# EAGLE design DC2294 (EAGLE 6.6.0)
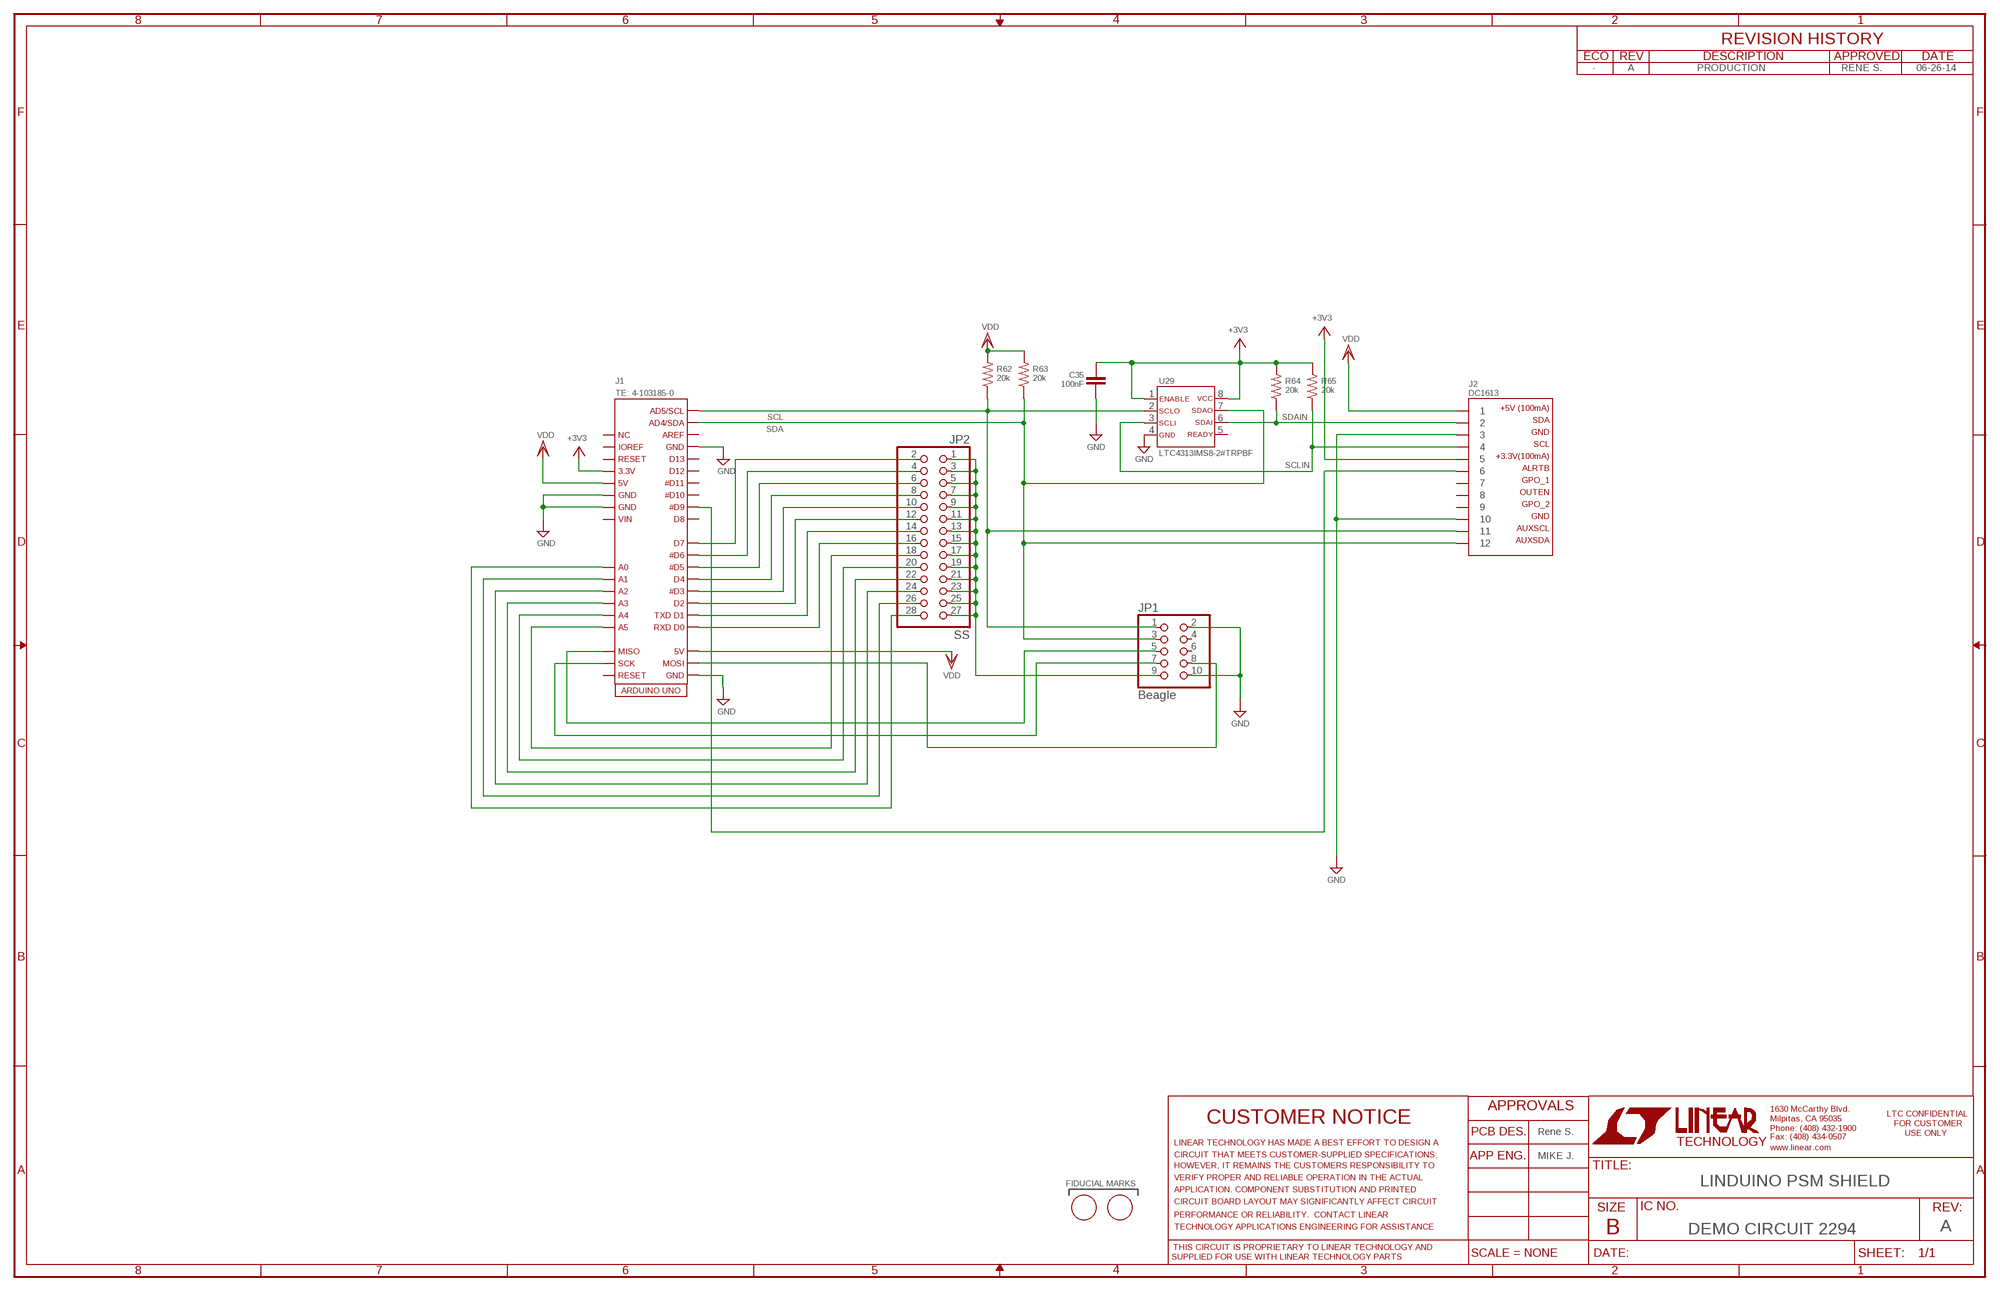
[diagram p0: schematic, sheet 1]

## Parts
C35  100nF  CC0603_BOX  [C0603_BOX]
FID1  FIDUCIAL  [FIDUCIAL_1MM]
FID2  FIDUCIAL  [FIDUCIAL_1MM]
J1  TE: 4-103185-0  ARDUINO_UNO_MINI_SHIELD_SPIFL  [ADRUINO_UNO_MINI_SHIELD_SPI_NOETH]
J2  DC1613  CONN_DC1613  [CONN_DC1613]
JP1  Beagle  PINHD-2X5  [2X05]
JP2  SS  PINHD-2X14  [2X14]
R62  20k  RR0603_BOX  [R0603_BOX]
R63  20k  RR0603_BOX  [R0603_BOX]
R64  20k  RR0603_BOX  [R0603_BOX]
R65  20k  RR0603_BOX  [R0603_BOX]
U29  LTC4313IMS8-2#TRPBF  LTC4313CMS8  [MSOP-8]

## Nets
+3V3: C35.1 J1.3V3 J2.5 R64.2 R65.2 U29.1 U29.8
GND: C35.2 J1.GND1 J1.GND2 J1.GND3 J1.GND4 J2.3 J2.10 JP1.2 JP1.10 U29.4
J1-A: J1.A0 JP2.28
N$1: J1.MISO JP1.5
N$2: J1.MOSI JP1.8
N$3: J1.SCK JP1.7
N$4: J1.D7 JP2.2
N$5: J1.D6 JP2.4
N$6: J1.D5 JP2.6
N$7: J1.D4 JP2.8
N$8: J1.D3 JP2.10
N$9: J1.D2 JP2.12
N$10: J1.D1 JP2.14
N$11: J1.D0 JP2.16
N$12: J1.A5 JP2.18
N$13: J1.A4 JP2.20
N$14: J1.A3 JP2.22
N$15: J1.A2 JP2.24
N$16: J1.A1 JP2.26
N$18: JP1.9 JP2.1 JP2.3 JP2.5 JP2.7 JP2.9 JP2.11 JP2.13 JP2.15 JP2.17 JP2.19 JP2.21 JP2.23 JP2.25 JP2.27
N$19: J1.D9 J2.6
SCL: J1.SCL J2.11 JP1.1 R62.1 U29.2
SCLIN: J2.4 R65.1 U29.3
SDA: J1.SDA J2.12 JP1.3 R63.1 U29.7
SDAIN: J2.2 R64.1 U29.6
VDD: J1.5V J1.5V1 J2.1 R62.2 R63.2
Unconnected: J1.D8 J1.D10 J1.D11 J1.D12 J1.D13 J1.NC J1.REF J1.RST1 J1.RST2 J1.VIN J1.VIO J2.7 J2.8 J2.9 JP1.4 JP1.6 U29.5

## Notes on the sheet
- A | PRODUCTION | RENE S. | 06-26-14
- Rene S.
- MIKE J.
- FIDUCIAL MARKS | LINDUINO PSM SHIELD
- DEMO CIRCUIT 2294 | A

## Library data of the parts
C35 = kalin:C: CAPACITOR, European symbol
FID1 FID2 = kalin:FIDUCIAL: For use by pick and place machines to calibrate the vision/machine, 1mm
J1 = kalin:ARDUINO_UNO_MINI_SHIELD_SPI: Arduino UNO Mini Shield With SPI
J2 = kalin:CONN_DC1613: Connector for LT DC1613 USB Dongle
JP1 = pinhead:PINHD-2X5: PIN HEADER
JP2 = pinhead:PINHD-2X14: PIN HEADER
R62-R65 = kalin:R: RESISTOR, American symbol
U29 = kalin:LTC4313: 2-Wire Bus Buffers with High Noise Margin

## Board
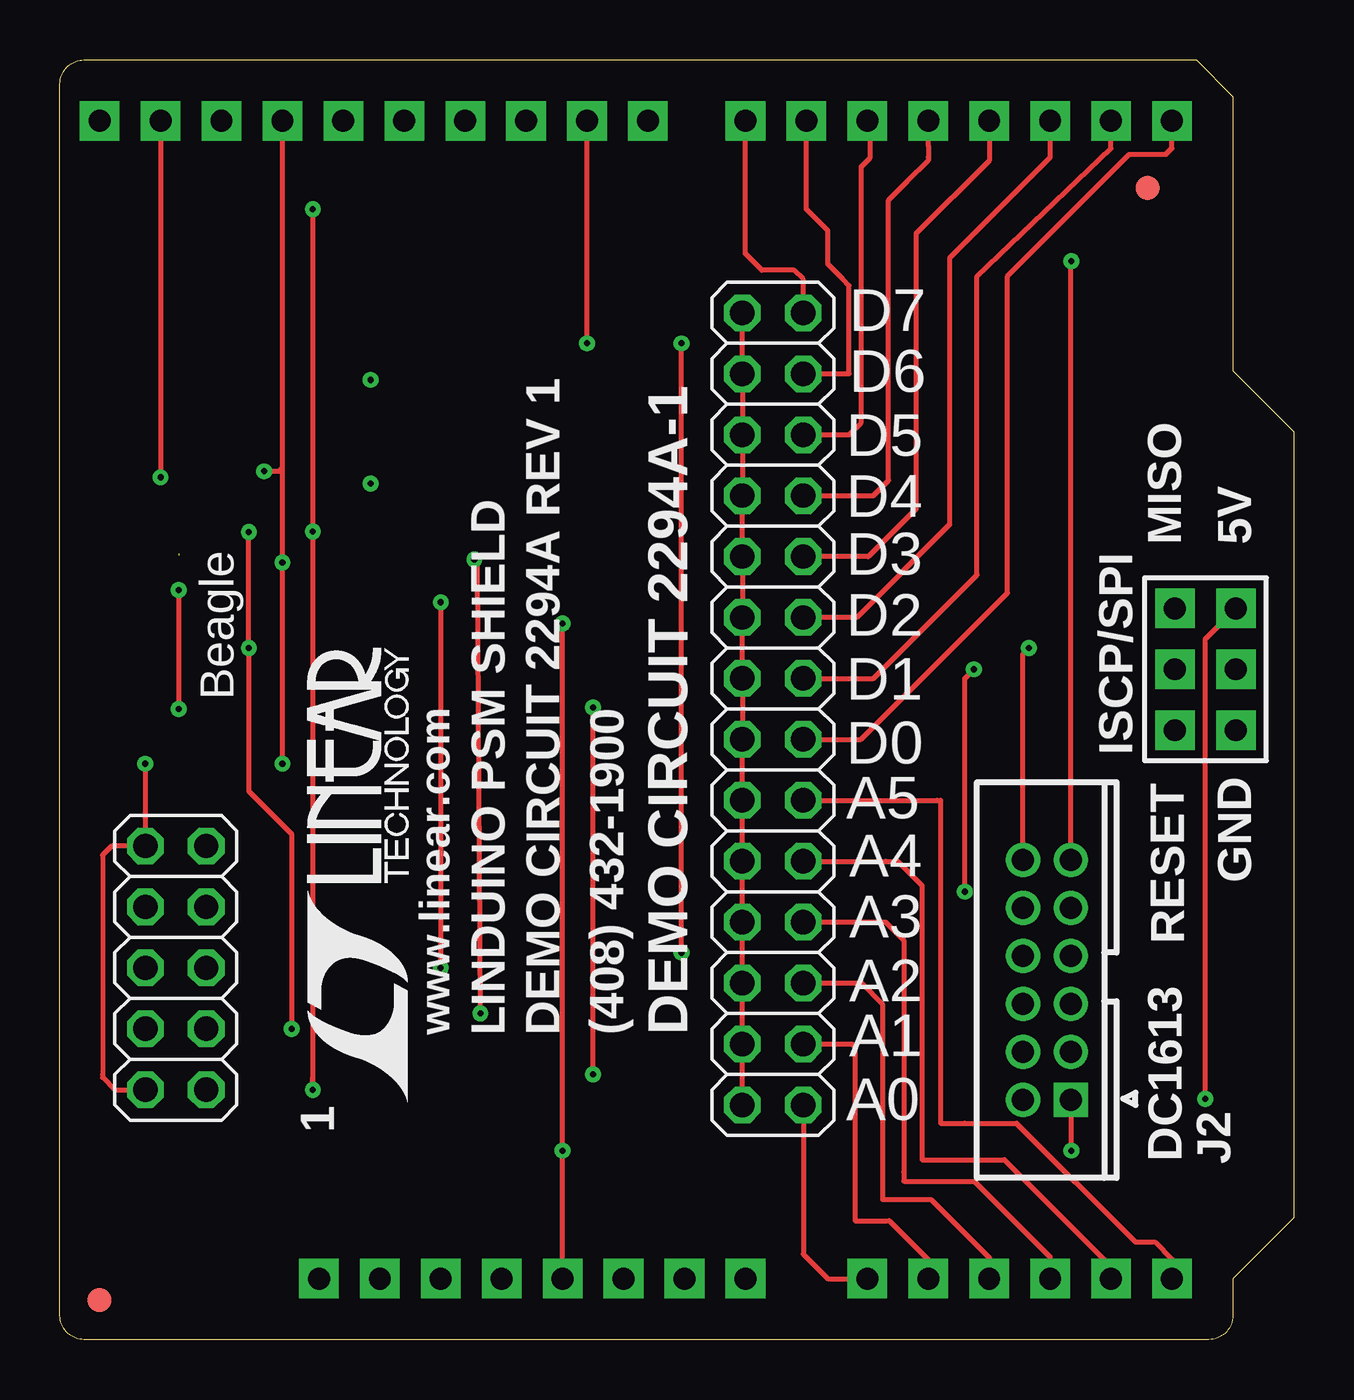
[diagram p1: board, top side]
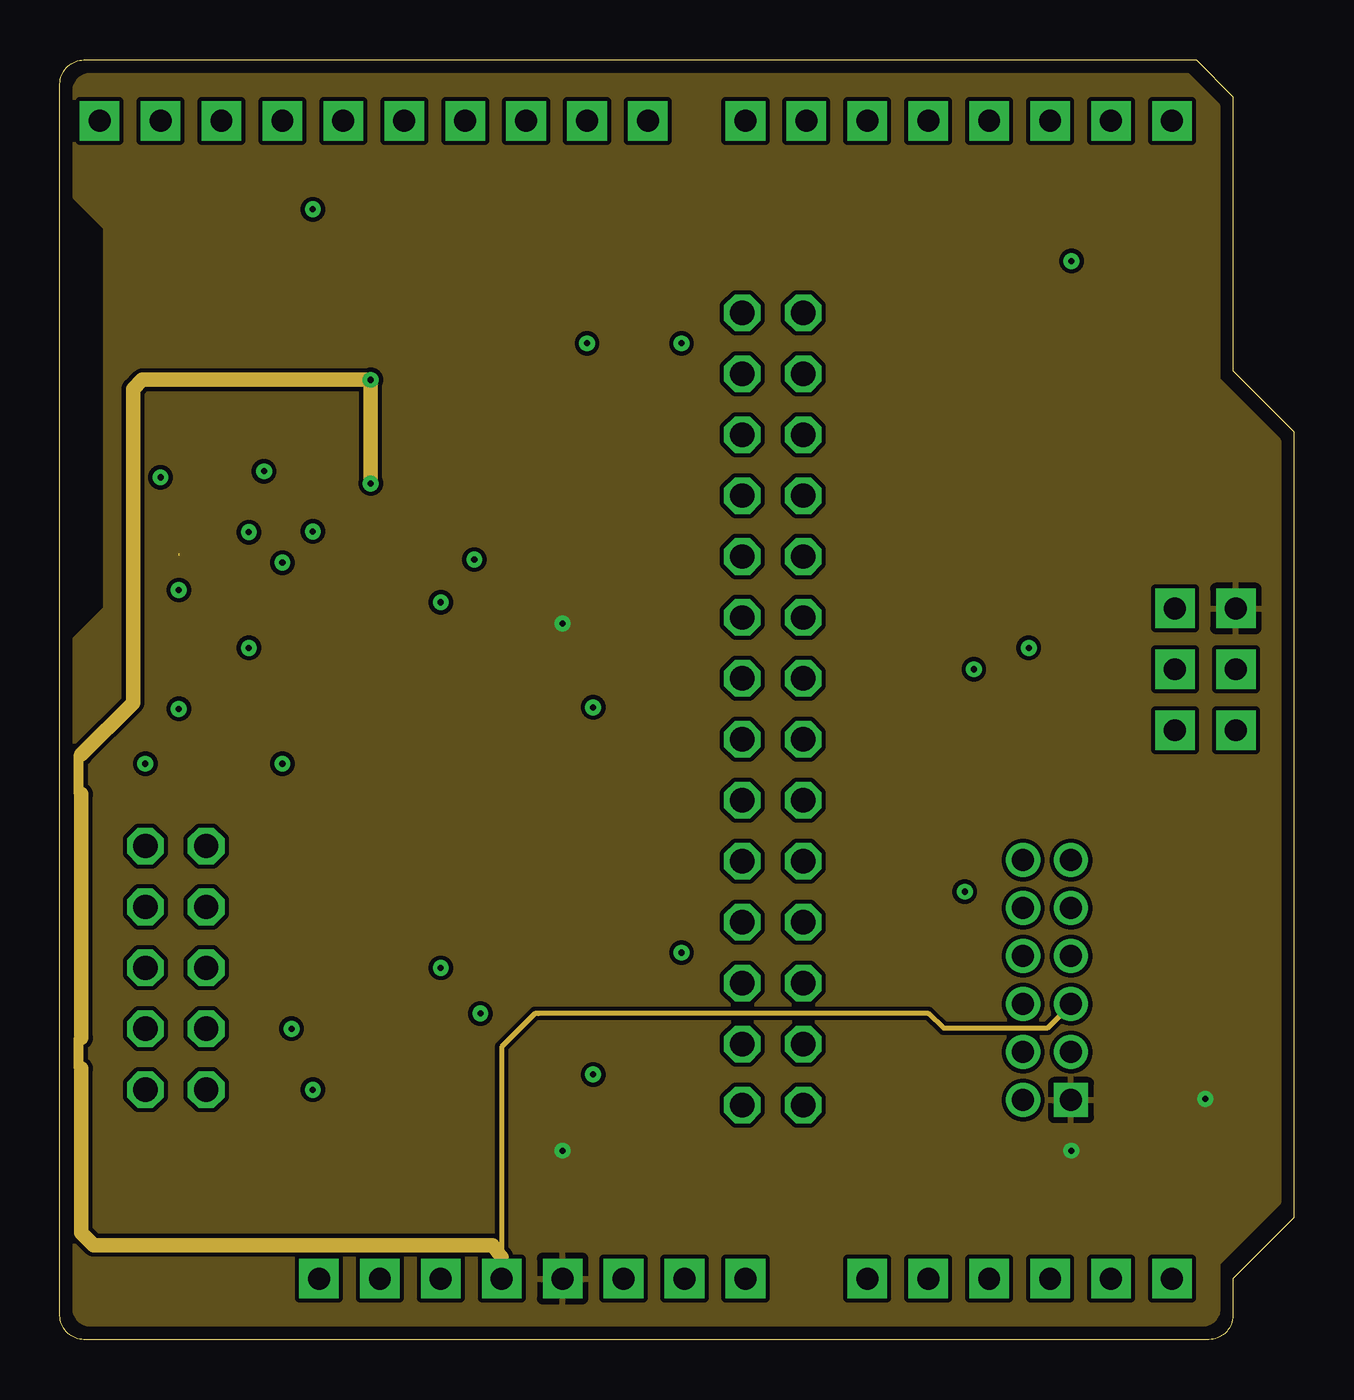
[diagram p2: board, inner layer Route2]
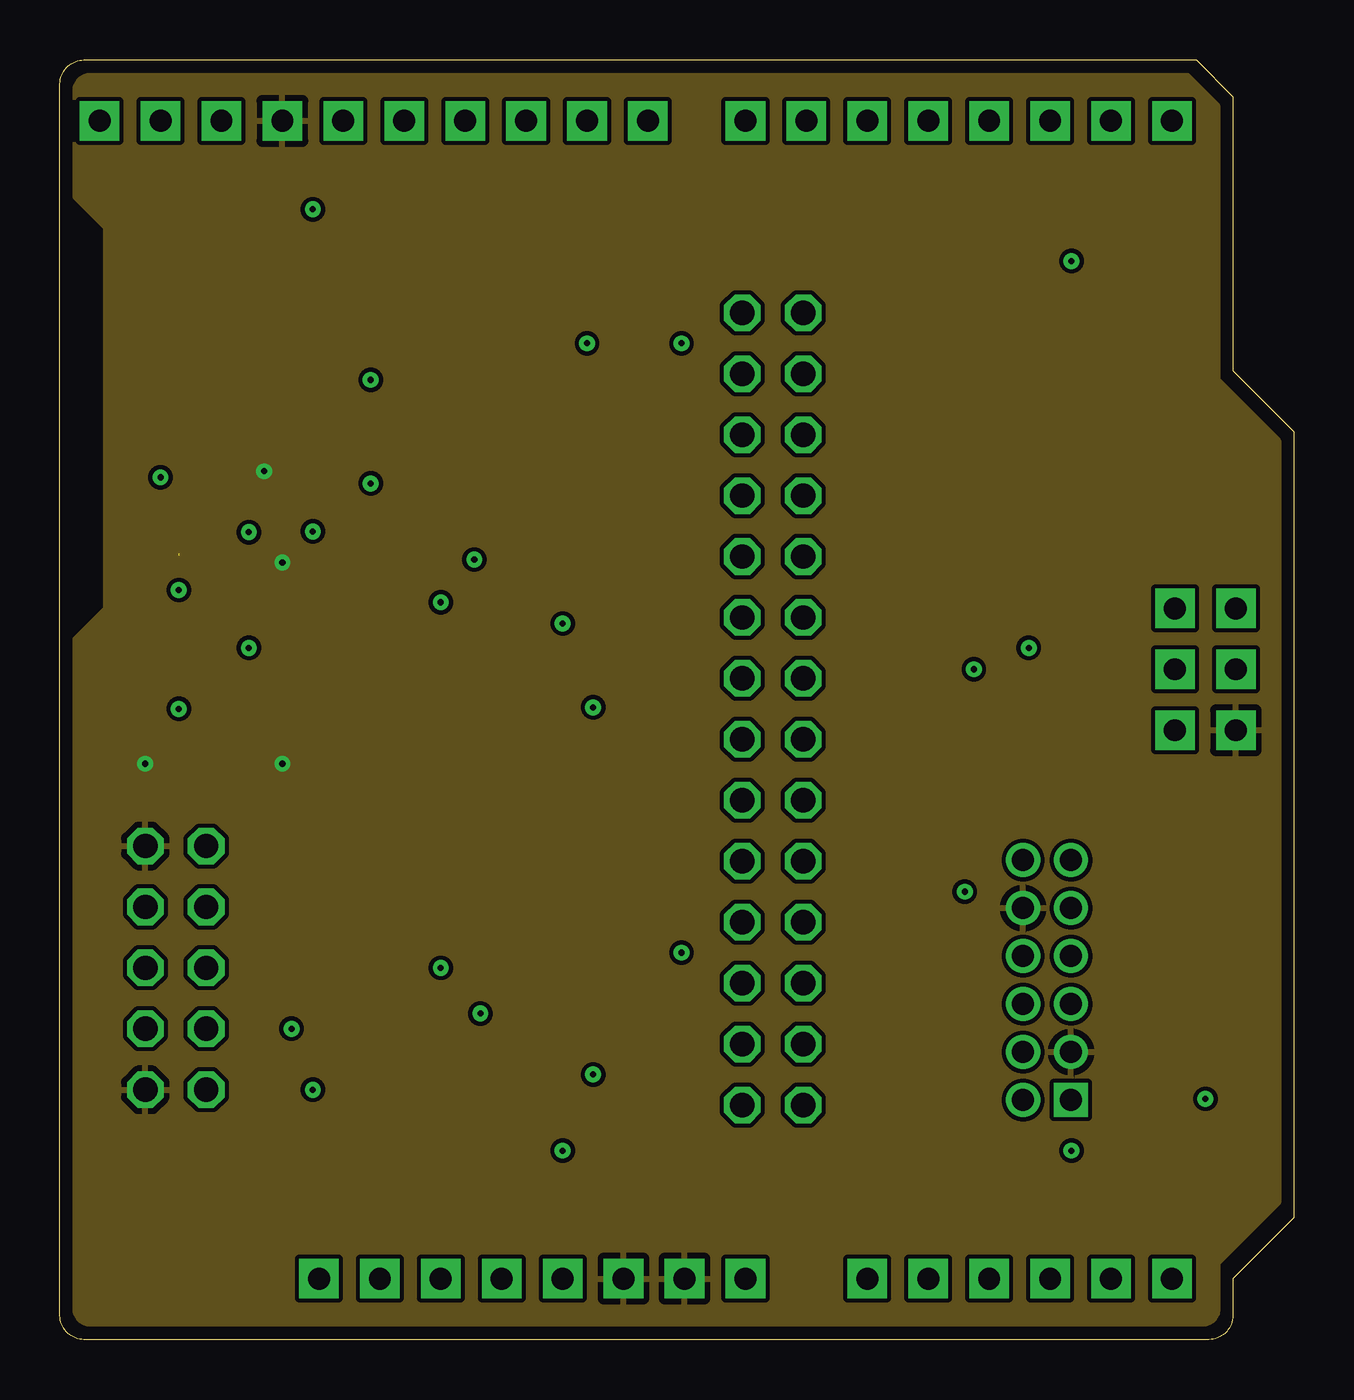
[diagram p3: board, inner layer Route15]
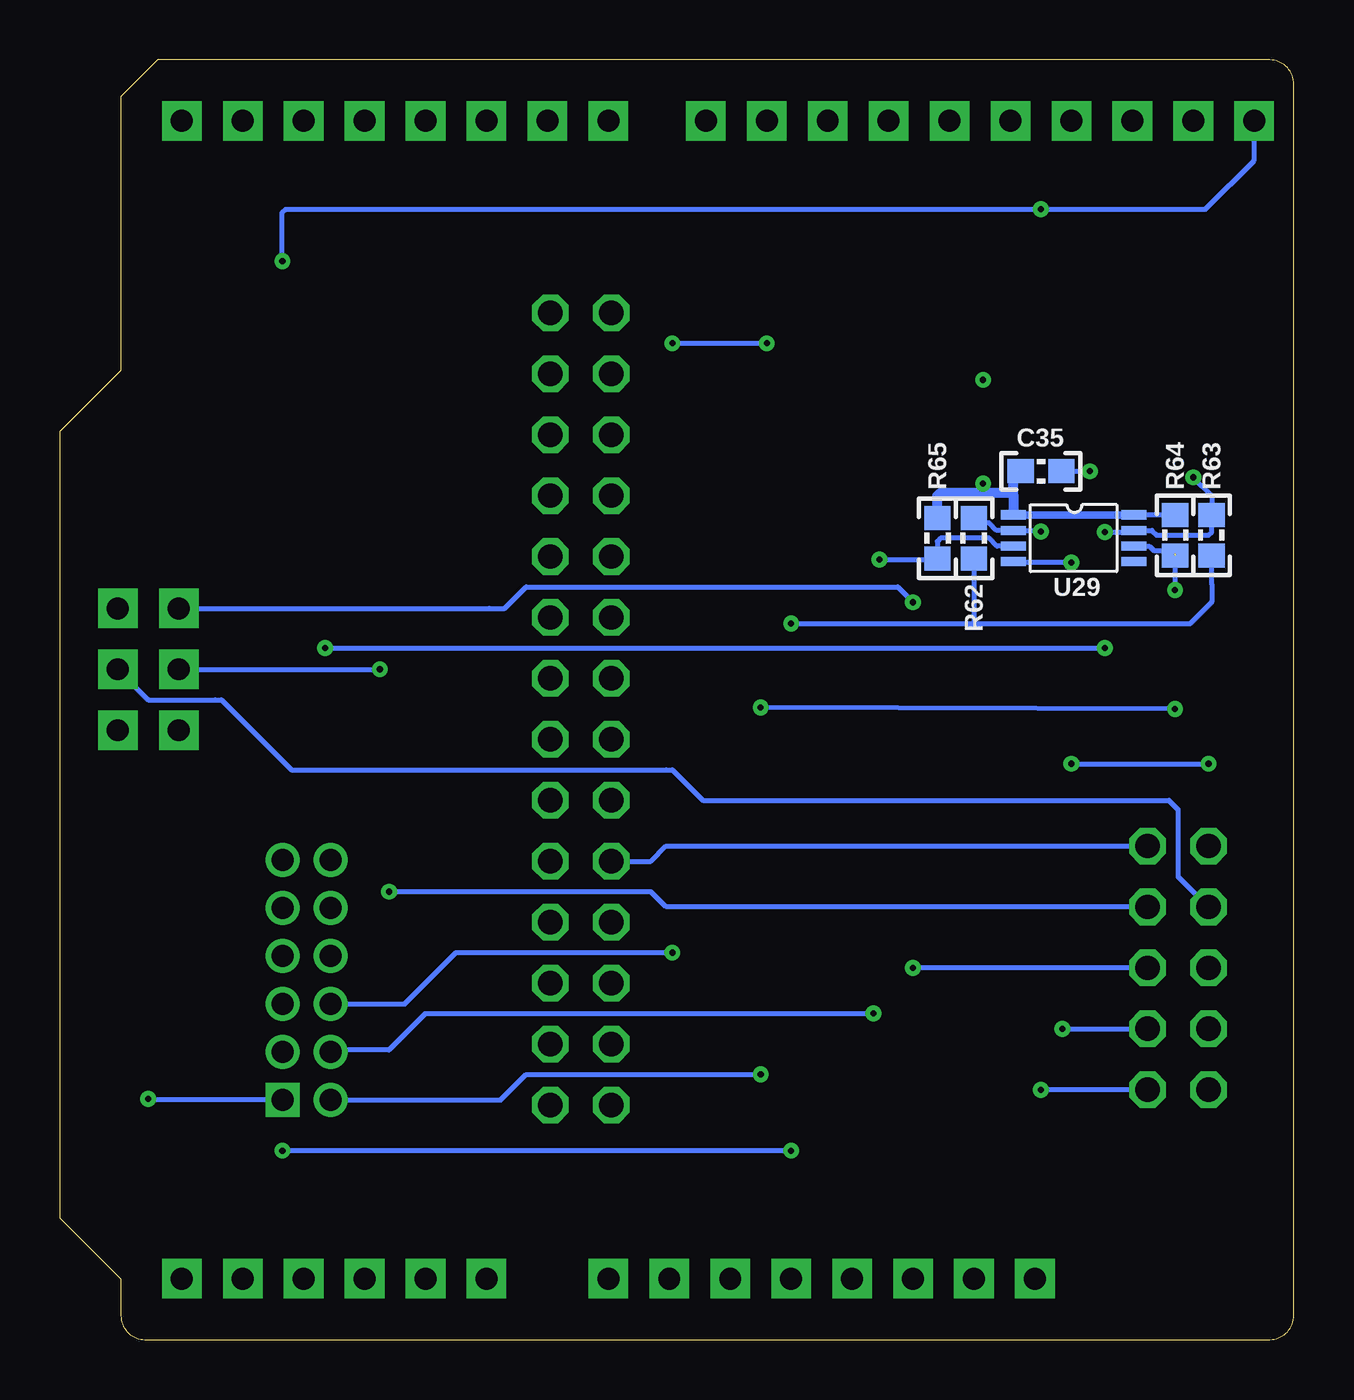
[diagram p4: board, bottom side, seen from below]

Size 51.44 x 53.34 mm. Coordinates in mm from the lower left corner, seen from the top.
Copper layers (1*2+15*16): Top 0.035mm / dielectric 1.5mm / Route2 0.035mm / dielectric 0.15mm / Route15 0.035mm / dielectric 0.2mm / Bottom 0.035mm
Design rules "default *": minimum track width 8mil, minimum drill 10mil, track to track 7mil, track to pad 7mil, pad to pad 7mil, via to via 7mil, smd to smd 1mil, copper to edge 20mil, drill to drill 15mil, minimum pad ring 10mil, minimum via ring 8mil, stop-mask expansion 4mil, vias tented up to drill 16mil, thermal gap 10mil

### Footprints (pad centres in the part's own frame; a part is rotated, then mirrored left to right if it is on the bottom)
C0603_BOX = smd 1.1 x 1: 1 -0.85,0; 2 0.85,0
FIDUCIAL_1MM = smd 1 x 1: 1 0,0
ADRUINO_UNO_MINI_SHIELD_SPI_NOETH = drill 0.914 pad 1.651 square: 3V3 18.415,2.54; 5V 20.955,2.54; 5V1 49.022,30.48; A0 33.655,2.54; A1 36.195,2.54; A2 38.735,2.54; A3 41.275,2.54; A4 43.815,2.54; A5 46.355,2.54; D0 46.355,50.8; D1 43.815,50.8; D2 41.275,50.8; D3 38.735,50.8; D4 36.195,50.8; D5 33.655,50.8; D6 31.115,50.8; D7 28.575,50.8; D8 24.511,50.8; D9 21.971,50.8; D10 19.431,50.8; D11 16.891,50.8; D12 14.351,50.8; D13 11.811,50.8; GND1 23.495,2.54; GND2 26.035,2.54; GND3 9.271,50.8; GND4 49.022,25.4; MISO 46.482,30.48; MOSI 49.022,27.94; NC 10.795,2.54; REF 6.731,50.8; RST1 15.875,2.54; RST2 46.482,25.4; SCK 46.482,27.94; SCL 1.651,50.8; SDA 4.191,50.8; VIN 28.575,2.54; VIO 13.335,2.54
CONN_DC1613 = drill 0.914 square: 1 -5,-1 | drill 0.914: 2 -5,1; 3 -3,-1; 4 -3,1; 5 -1,-1; 6 -1,1; 7 1,-1; 8 1,1; 9 3,-1; 10 3,1; 11 5,-1; 12 5,1
2X05 = drill 1.016 octagon: 1 -5.08,-1.27; 2 -5.08,1.27; 3 -2.54,-1.27; 4 -2.54,1.27; 5 0,-1.27; 6 0,1.27; 7 2.54,-1.27; 8 2.54,1.27; 9 5.08,-1.27; 10 5.08,1.27
2X14 = drill 1.016 octagon: 1 -16.51,-1.27; 2 -16.51,1.27; 3 -13.97,-1.27; 4 -13.97,1.27; 5 -11.43,-1.27; 6 -11.43,1.27; 7 -8.89,-1.27; 8 -8.89,1.27; 9 -6.35,-1.27; 10 -6.35,1.27; 11 -3.81,-1.27; 12 -3.81,1.27; 13 -1.27,-1.27; 14 -1.27,1.27; 15 1.27,-1.27; 16 1.27,1.27; 17 3.81,-1.27; 18 3.81,1.27; 19 6.35,-1.27; 20 6.35,1.27; 21 8.89,-1.27; 22 8.89,1.27; 23 11.43,-1.27; 24 11.43,1.27; 25 13.97,-1.27; 26 13.97,1.27; 27 16.51,-1.27; 28 16.51,1.27
R0603_BOX = smd 1 x 1.1: 1 -0.85,0; 2 0.85,0
MSOP-8 = smd 1.041 x 0.381: 1 -2.55,0.975; 2 -2.55,0.325; 3 -2.55,-0.325; 4 -2.55,-0.975; 5 2.479,-0.975; 6 2.479,-0.325; 7 2.479,0.325; 8 2.479,0.975

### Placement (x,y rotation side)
C35  10.54,36.2 0 bottom
DRILEGEND  [DRILEGEND]  not placed on the board
FID1  45.34,48.01 0 top
FID2  1.65,1.65 0 top
J1  0,0 0 top
J2  41.15,14.99 90 top
JP1  4.83,15.49 90 top
JP2  29.72,26.29 270 top
R62  13.34,33.4 270 bottom
R63  3.43,33.53 270 bottom
R64  4.95,33.53 90 bottom
R65  14.86,33.4 90 bottom
U29  9.14,33.4 0 bottom
U$3  [DC2294_FRAME]  not placed on the board
U$5  [LT_LOGO_LARGE_SILK]  14.61,9.78 90 top

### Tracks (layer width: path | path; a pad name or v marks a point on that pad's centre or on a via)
+3V3  (via drill 0.25)
  Route2 0.203: J2.5 42.15,13.95 41.16,12.98 36.84,12.98 36.2,13.59 19.94,13.59 19.81,13.59 18.41,12.19 J1.3V3
  Route2 0.406: 0.89,11.3 0.79,11.3 0.79,12.57 0.89,12.57 | 0.89,22.73 0.79,22.73 0.79,24.38 0.89,24.38
  Route2 0.61: J1.3V3 18.41,3.43 18.03,3.94 1.4,3.94 0.89,4.45 0.89,11.3 | 0.89,12.57 0.89,22.73 | 0.89,24.38 3.05,26.54 3.05,39.62 3.43,40.01 v12.95,40.01 v12.95,35.69
  Bottom 0.203: U29.1 | R64.2 U29.8 | 14.9,34.29 R65.2
  Bottom 0.305: U29.1 U29.8
  Bottom 0.406: R65.2 14.86,35.18 14.73,35.31 12.95,35.31 | 12.95,35.31 11.81,35.31 11.68,35.18 | 11.68,35.18 U29.1 | 12.95,35.31 v12.95,35.69 | 11.68,35.18 11.68,36.16 C35.1
GND  (via drill 0.25 pad 0.25)
  Top 0.203: JP1.2 2.29,10.41 1.78,10.92 1.78,11.05 1.78,20.19 2.16,20.57 JP1.10 v3.56,24 | J1.GND3 9.27,37.47 9.27,36.32 | 9.27,36.32 v9.27,32.38 v9.27,24 | v8.51,36.2 9.14,36.2 9.27,36.32
  Bottom 0.203: v9.27,32.38 11.65,32.38 U29.4 | C35.2 v8.51,36.2 | v9.27,24 v3.56,24
  pour Route15 (rank 6): 1.27,52.7 46.99,52.7 48.26,51.44 48.26,40.01 50.8,37.47 50.8,5.71 48.26,3.17 48.26,1.27 arc-90 47.62,0.64 1.27,0.64 arc-90 0.64,1.27 0.64,29.21 1.91,30.48 1.91,46.35 0.64,47.62 0.64,52.07 arc-90
J1-A
  Top 0.203: JP2.28 30.99,3.56 32,2.54 J1.A0
N$1  (via drill 0.25)
  Top 0.203: v15.88,30.73 v15.88,15.49
  Bottom 0.203: JP1.5 15.62,15.49 | 15.62,15.49 v15.88,15.49 15.62,15.49 | J1.MISO 33.53,30.48 32.89,30.48 32,31.37 16.51,31.37 v15.88,30.73
N$2
  Bottom 0.203: J1.MOSI 47.75,26.67 44.96,26.67 44.7,26.67 41.78,23.75 26.16,23.75 25.91,23.75 24.64,22.48 5.21,22.48 4.83,22.1 4.83,19.3 JP1.8
N$3  (via drill 0.25 pad 0.25)
  Top 0.203: v37.72,18.67 37.72,27.56 v38.1,27.94
  Bottom 0.203: JP1.7 26.16,18.03 26.8,18.67 v37.72,18.67 | J1.SCK v38.1,27.94
N$4
  Top 0.203: JP2.2 30.99,44.2 30.61,44.58 29.26,44.58 28.57,45.26 28.57,46.99 J1.D7
N$5
  Top 0.203: JP2.4 32.89,40.26 32.89,43.94 32.64,44.2 32,44.83 32,46.23 31.11,47.12 J1.D6
N$6
  Top 0.203: JP2.6 32.26,37.72 32.89,37.72 33.4,38.23 33.4,48.64 33.4,48.9 33.78,49.28 33.78,50.67 J1.D5
N$7
  Top 0.203: JP2.8 32.89,35.18 33.91,35.18 34.54,35.81 34.54,47.5 35.31,48.26 36.2,49.15 36.2,49.28 36.2,49.78 J1.D4
N$8
  Top 0.203: J1.D3 38.73,49.15 35.69,46.1 35.69,35.05 35.69,34.63 33.7,32.64 JP2.10
N$9
  Top 0.203: JP2.12 33.21,30.1 37.08,33.97 37.08,45.09 41.15,49.15 41.27,49.28 J1.D2
N$10
  Top 0.203: JP2.14 33.92,27.56 38.23,31.87 38.23,44.32 43.81,49.66 J1.D1
N$11
  Top 0.203: JP2.16 33.39,25.02 39.5,31.13 39.5,44.32 39.62,44.45 44.58,49.4 45.97,49.4 46.1,49.4 46.35,49.66 J1.D0
N$12
  Top 0.203: JP2.18 36.58,22.48 36.7,22.48 36.7,21.34 36.7,9.02 37.72,9.02 39.88,9.02 44.83,4.06 45.64,4.06 46.35,3.35 J1.A5
N$13
  Top 0.203: JP2.20 34.42,19.94 34.92,19.94 35.94,18.92 35.94,7.49 39.37,7.49 43.81,3.05 J1.A4
N$14
  Top 0.203: JP2.22 34.29,17.4 34.42,17.4 35.18,16.64 35.18,6.99 35.18,6.6 38.12,6.6 41.27,3.45 J1.A3
N$15
  Top 0.203: JP2.24 33.27,14.86 33.4,14.86 34.29,13.97 34.29,6.48 34.29,5.84 36.31,5.84 38.73,3.42 J1.A2
N$16
  Top 0.203: JP2.26 33.02,12.32 33.15,12.19 33.15,5.71 33.15,4.95 34.57,4.95 36.2,3.33 J1.A1
N$18
  Top 0.203: JP2.1 JP2.3 JP2.5 JP2.7 JP2.9 JP2.11 JP2.13 JP2.15 JP2.17 JP2.19 JP2.21 JP2.23 JP2.25 JP2.27
  Bottom 0.203: JP2.19 26.8,19.94 26.16,20.57 JP1.9
N$19  (via drill 0.25, 0.25 pad 0.25)
  Top 0.203: v21.97,41.53 J1.D9 | v25.91,16.13 v25.91,41.53
  Bottom 0.203: J2.6 37.07,13.99 34.92,16.13 v25.91,16.13 | v25.91,41.53 24.13,41.53 v21.97,41.53
SCL  (via drill 0.25, 0.25 pad 0.25)
  Top 0.203: 10.54,10.92 v10.54,33.69 v10.54,47.12 | 10.54,10.92 v10.54,10.41 10.54,10.92 | J2.11 42.15,44.94 v42.16,44.96
  Bottom 0.203: R62.1 13.34,34.04 12.7,34.04 12.39,33.73 U29.2 10.54,33.72 | v10.54,47.12 42.04,47.12 42.16,46.99 v42.16,44.96 | v10.54,47.12 10.41,47.12 | 10.41,47.12 3.68,47.12 1.65,49.15 J1.SCL | 10.54,33.72 10.55,33.72 10.54,33.72 | 10.54,33.72 10.54,33.73 v10.54,33.69 | v10.54,47.12 10.41,47.12 | JP1.1 v10.54,10.41
SCLIN  (via drill 0.25 pad 0.25)
  Top 0.203: v17.53,13.59 17.4,32.38 v17.27,32.51
  Bottom 0.203: U29.3 12.38,33.08 12.7,33.4 14.73,33.4 14.86,33.27 R65.1 14.9,32.51 17.14,32.51 | 17.4,32.51 v17.27,32.51 | v17.27,32.51 17.14,32.51 | v17.53,13.59 36.2,13.59 37.72,12.06 40.07,12.06 J2.4 | v17.27,32.51 17.14,32.51
SDA  (via drill 0.25, 0.25 pad 0.25)
  Top 0.203: v7.87,33.66 v7.87,28.83 7.87,22.86 9.65,21.08 v9.65,12.95 | J1.SDA v4.19,35.94 | J2.12 40.15,28.59 v40.39,28.83
  Bottom 0.203: R63.1 3.43,33.66 3.56,33.53 5.71,33.53 5.91,33.73 U29.7 6.74,33.66 v7.87,33.66 | 3.43,34.29 R63.1 | 3.43,34.42 R63.1 | v40.39,28.83 v7.87,28.83 | v4.19,35.94 3.43,35.18 R63.1 | v9.65,12.95 JP1.3
SDAIN  (via drill 0.25, 0.25 pad 0.25)  (1 unrouted)
  Top 0.203: v4.95,31.24 v4.95,26.29 | v22.23,11.05 v22.23,26.35 | v22.23,26.35
  Bottom 0.203: U29.6 6.03,33.08 5.84,32.89 5.17,32.89 R64.1 | 4.95,32.77 v4.95,31.24 | v4.95,26.29 v22.23,26.35 | v22.23,26.35 22.1,26.35 22.35,26.35 v22.23,26.35 | J2.2 33.07,9.99 32,11.05 v22.23,11.05
VDD  (via drill 0.25, 0.25 pad 0.25)
  Top 0.203: J1.5V v20.95,7.87 v20.95,29.84 | v47.75,10.03 47.75,29.21 J1.5V1 | v42.16,7.87 42.16,9.97 J2.1
  Bottom 0.203: v20.95,29.84 13.34,29.84 | 13.34,29.84 13.21,29.84 4.32,29.84 3.43,30.73 3.43,31.5 R63.2 | R62.2 13.34,32.51 13.34,32.38 13.34,29.84 | J2.1 47.75,9.99 v47.75,10.03 | v20.95,7.87 v42.16,7.87
  pour Route2 (rank 6): 1.27,52.7 46.99,52.7 48.26,51.44 48.26,40.01 50.8,37.47 50.8,5.71 48.26,3.17 48.26,1.27 arc-90 47.62,0.64 1.27,0.64 arc-90 0.64,1.27 0.64,29.21 1.91,30.48 1.91,46.35 0.64,47.62 0.64,52.07 arc-90

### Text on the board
tPlace: D7 | D6 | D5 | D4 | MISO | 5V | D3 | D2 | D1 | D0 | ISCP/SPI | A5 | A4 | GND | A3 | RESET | A2 | www.linear.com | LINDUINO PSM SHIELD | DEMO CIRCUIT 2294A REV 1 | (408) 432-1900 | DEMO CIRCUIT 2294A-1 | A1 | 1 | A0
d_FabDrawing: DRILL TABLE
DrillLegend_01-16: 01-16
DrillLegend: LAYER-STACK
